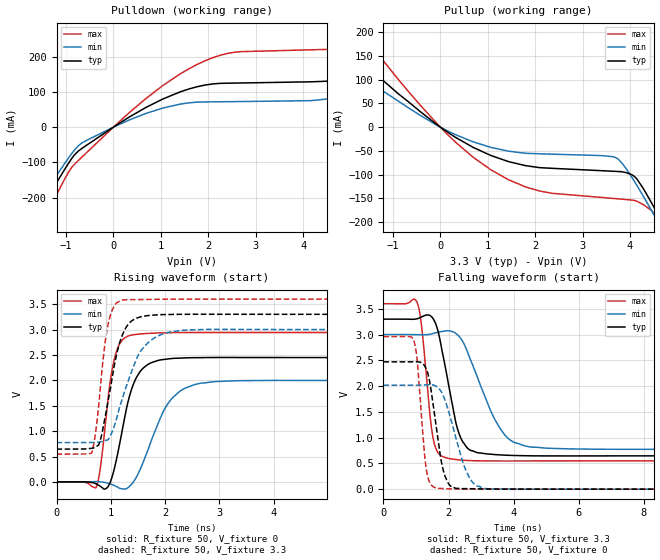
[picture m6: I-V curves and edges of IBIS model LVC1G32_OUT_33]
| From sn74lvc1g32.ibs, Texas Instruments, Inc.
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[Model]   LVC1G32_OUT_33
Model_type  Output
Vref =   0.0
Rref =   500
Cref =   50p
Vmeas =   1.5
| variable   typ   min   max
C_comp   8.24pF   3.83pF   13.13pF
| C_pullup   7.22pF   3.83pF   8.98pF
| C_pulldown   9.27pF   5.75pF   13.13pF
[Temperature Range]   40   100   -40
| Ambient temperature   25   85   -40
[Voltage range]   3.3   3   3.6
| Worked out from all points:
|   slope of the pulldown table from 0 to 0.495 V, typ, clamps not added: 12 ohm
|   slope of the pullup table from 0 to 0.495 V, typ, clamps not added: 15.7 ohm
|   rising waveform, R_fixture 50, V_fixture 0: 20-80 % time 316ps typ, 489ps min, 207ps max; typ from 0 V to 2.45 V
|   rising waveform, R_fixture 50, V_fixture 3.3: 20-80 % time 295ps typ, 439ps min, 189ps max; typ from 0.647 V to 3.3 V
|   falling waveform, R_fixture 50, V_fixture 3.3: 20-80 % time 497ps typ, 898ps min, 282ps max; typ from 3.3 V to 0.647 V
|   falling waveform, R_fixture 50, V_fixture 0: 20-80 % time 343ps typ, 558ps min, 219ps max; typ from 2.47 V to 0 V
[Pulldown]
| LVC1G32_OUT_33
|   Voltage   I(typ)   I(min)   I(max)
-5V       -1.007A    -902.2mA   -1.174A
-2.465V   -446.6mA   -395.8mA   -527.8mA
-1.49V    -223.7mA   -195.8mA   -268.8mA
-565mV    -51.17mA   -37.44mA   -72.18mA
1.045V    80.07mA    54.27mA    118.3mA
2.25V     124.2mA    72mA       203.9mA
4.955V    139mA      90.75mA    224.3mA
6.94V     245.6mA    179.1mA    349.1mA
7.53V     288.8mA    86.31mA    407.3mA
7.915V    302.5mA    81.48mA    448.3mA
8.75V     158mA      82.48mA    511mA
10V       144.3mA    84.07mA    276.2mA
[Pullup]
| LVC1G32_OUT_33
|   Voltage   I(typ)   I(min)   I(max)
-5V       498.4mA    400.8mA    691mA
-3.33V    311.1mA    247mA      435.1mA
-2.555V   229.2mA    180.5mA    322.4mA
-1.88V    161.5mA    126mA      228.6mA
-70mV     5.134mA    3.851mA    7.467mA
1.065V    -59.73mA   -42.64mA   -89.86mA
2.1V      -85.39mA   -56.25mA   -134.8mA
3.66V     -93.08mA   -62.51mA   -150.4mA
4.145V    -109.4mA   -122.9mA   -156.2mA
4.63V     -192.2mA   -207.1mA   -202.9mA
4.77V     -218.8mA   -232.4mA   -230.8mA
10V       -1.305A    -1.242A    -1.439A
[Ramp]
| LVC1G32_OUT_33
| variable   typ   min   max
dV/dt_r   1.56/3.30E-10   1.28/5.44E-10   1.84/2.17E-10
dV/dt_f   1.64/5.40E-10   1.38/9.55E-10   1.89/2.95E-10
R_load = 50
[Rising Waveform]
| LVC1G32_OUT_33
R_fixture =   50
C_fixture =   0
L_fixture =   0
V_fixture =   0
V_fixture_min = 0
V_fixture_max = 0
|   Time   V(typ)   V(min)   V(max)
0s        -33.62uV   -68.5uV    -10.33uV
725ps     -35.37mV   6.197mV    -115.5mV
810ps     -88.36mV   1.223mV    296.9mV
945ps     -99.65mV   -23.7mV    1.591V
1.165ns   764.2mV    -126.6mV   2.722V
1.4ns     1.878V     -22.33mV   2.895V
1.7ns     2.324V     675.9mV    2.925V
2.27ns    2.437V     1.782V     2.941V
3.325ns   2.45V      1.993V     2.943V
50ns      2.447V     1.995V     2.942V
[Rising Waveform]
| LVC1G32_OUT_33
R_fixture =   50
C_fixture =   0
L_fixture =   0
V_fixture =   3.3
V_fixture_min = 3
V_fixture_max = 3.6
|   Time   V(typ)   V(min)   V(max)
0s        646.7mV    774.3mV    548mV
645ps     661.9mV    776.8mV    567.9mV
790ps     766.7mV    785.7mV    1.652V
960ps     1.654V     845.1mV    3.146V
1.135ns   2.634V     1.362V     3.546V
1.31ns    3.088V     1.957V     3.59V
1.525ns   3.242V     2.535V     3.591V
1.785ns   3.285V     2.823V     3.595V
2.75ns    3.301V     3.003V     3.6V
50ns      3.3V       3V         3.6V
[Falling Waveform]
| LVC1G32_OUT_33
R_fixture =   50
C_fixture =   0
L_fixture =   0
V_fixture =   3.3
V_fixture_min = 3
V_fixture_max = 3.6
|   Time   V(typ)   V(min)   V(max)
0s        3.3V       3V         3.6V
1.045ns   3.309V     2.998V     3.605V
1.17ns    3.343V     2.996V     3.171V
1.525ns   3.309V     3.021V     992.2mV
1.76ns    2.825V     3.056V     652.7mV
2.32ns    1.083V     2.967V     567.6mV
2.66ns    757.6mV    2.533V     554.1mV
3.6ns     664.1mV    1.162V     546.5mV
4.58ns    646.6mV    813.6mV    547.1mV
50ns      646.7mV    774.3mV    548mV
[Falling Waveform]
| LVC1G32_OUT_33
R_fixture =   50
C_fixture =   0
L_fixture =   0
V_fixture =   0
V_fixture_min = 0
V_fixture_max = 0
|   Time   V(typ)   V(min)   V(max)
0s        2.471V     2.018V     2.961V
935ps     2.472V     2.018V     2.881V
1.04ns    2.472V     2.019V     2.478V
1.32ns    2.324V     2.024V     373.7mV
1.685ns   929.7mV    1.963V     16.8mV
1.845ns   350.8mV    1.804V     10.11mV
2.045ns   69.05mV    1.417V     6.345mV
2.605ns   8.863mV    266.7mV    892uV
3.185ns   3.067mV    7.577mV    -380uV
50ns      -31.76uV   -65.2uV    -6.017uV
